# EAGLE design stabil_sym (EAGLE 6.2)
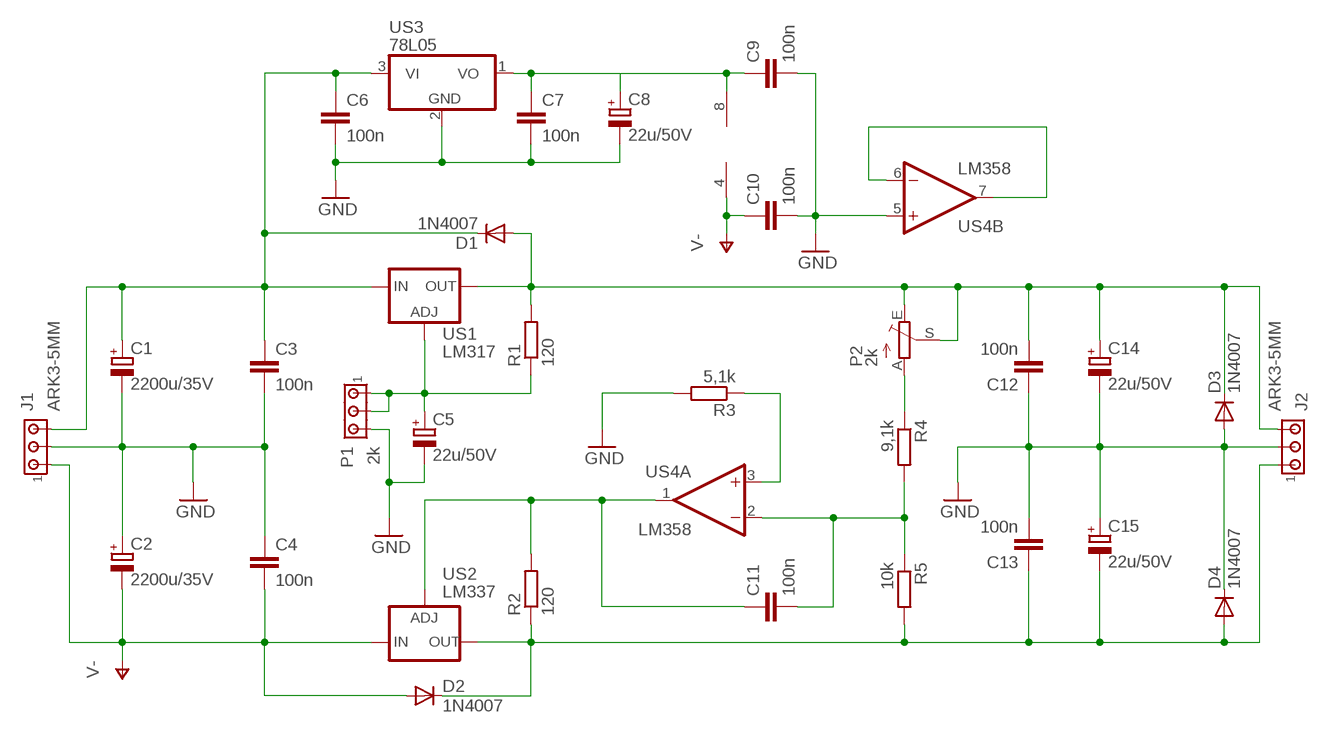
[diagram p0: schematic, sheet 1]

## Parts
C1  2200u/35V  CPOL-EUE7.5-18  [E7,5-18]
C2  2200u/35V  CPOL-EUE7.5-18  [E7,5-18]
C3  100n  C-EU050-025X075  [C050-025X075]
C4  100n  C-EU050-025X075  [C050-025X075]
C5  22u/50V  CPOL-EUE2.5-6  [E2,5-6]
C6  100n  C-EU050-025X075  [C050-025X075]
C7  100n  C-EU050-025X075  [C050-025X075]
C8  22u/50V  CPOL-EUE2.5-6  [E2,5-6]
C9  100n  C-EU050-025X075  [C050-025X075]
C10  100n  C-EU050-025X075  [C050-025X075]
C11  100n  C-EU050-025X075  [C050-025X075]
C12  100n  C-EU050-025X075  [C050-025X075]
C13  100n  C-EU050-025X075  [C050-025X075]
C14  22u/50V  CPOL-EUE2.5-6  [E2,5-6]
C15  22u/50V  CPOL-EUE2.5-6  [E2,5-6]
D1  1N4007  1N4004  [DO41-10]
D2  1N4007  1N4004  [DO41-10]
D3  1N4007  1N4004  [DO41-10]
D4  1N4007  1N4004  [DO41-10]
J1  ARK3-5MM  [3PIN-5MM]
J2  ARK3-5MM  [3PIN-5MM]
P1  2k  ARK3-5MM  [3PIN-5MM]
P2  2k  TRIM_EU-B64Y  [B64Y]
R1  120  R-EU_0207/7  [0207/7]
R2  120  R-EU_0207/7  [0207/7]
R3  5,1k  R-EU_0207/7  [0207/7]
R4  9,1k  R-EU_0207/7  [0207/7]
R5  10k  R-EU_0207/7  [0207/7]
US1  LM317  LM317TS  [317TS]
US2  LM337  LM337TS  [337TS]
US3  78L05  7805L  [TO92]
US4  LM358  LM358N  [DIL08]

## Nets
GND: C1.- C2.+ C3.2 C4.1 C5.- C6.2 C7.2 C8.- C9.2 C10.2 C12.1 C13.2 C14.- C15.+ D3.A D4.C J1.P$2 J2.P$2 P1.P$3 R3.2 US3.2(GND) US4.5(B:+IN)
N$1: C1.+ C3.1 C6.1 D1.C J1.P$3 US1.3(IN) US3.3(VI)
N$2: R3.1 US4.3(A:+IN)
N$3: P2.A R4.1
N$4: C12.2 C14.+ D1.A D3.C J2.P$3 P2.E P2.S R1.2 US1.2(OUT)
N$5: C13.1 C15.- D2.C D4.A J2.P$1 R2.1 R5.2 US2.3(OUT)
N$6: C5.+ P1.P$1 P1.P$2 R1.1 US1.1(ADJ)
N$7: C11.1 R2.2 US2.1(ADJ) US4.1(A:OUT)
N$8: C11.2 R4.2 R5.1 US4.2(A:-IN)
N$9: C7.1 C8.+ C9.1 US3.1(VO) US4.8(P:V+)
N$10: US4.6(B:-IN) US4.7(B:OUT)
V-: C2.- C4.2 C10.1 D2.A J1.P$1 US2.2(IN) US4.4(P:V-)

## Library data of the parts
C1 C2 C5 C8 C14 C15 = rcl:CPOL-EU: POLARIZED CAPACITOR, European symbol
C3 C4 C6 C7 C9-C13 = rcl:C-EU: CAPACITOR, European symbol
D1-D4 = diode:1N4004: DIODE
J1 J2 P1 = zlacza_futrzak:ARK3: ARK 3 Raster 5mm i 3,5mm
P2 = pot:TRIM_EU-: POTENTIOMETER
R1-R5 = rcl:R-EU_: RESISTOR, European symbol
US1 = v-reg:LM317TS: VOLTAGE REGULATOR
US2 = v-reg:LM337TS: VOLTAGE REGULATOR
US3 = linear:78*: Positive VOLTAGE REGULATOR Source: http://cache.national.com/ds/LM/LM78L05.pdf http://www.fairchildsemi.com/ds/LM/LM7805.pdf
US4 = linear:LM358: OP AMP also LM158; LM258; LM2904 Source: http://cache.national.com/ds/LM/LM158.pdf

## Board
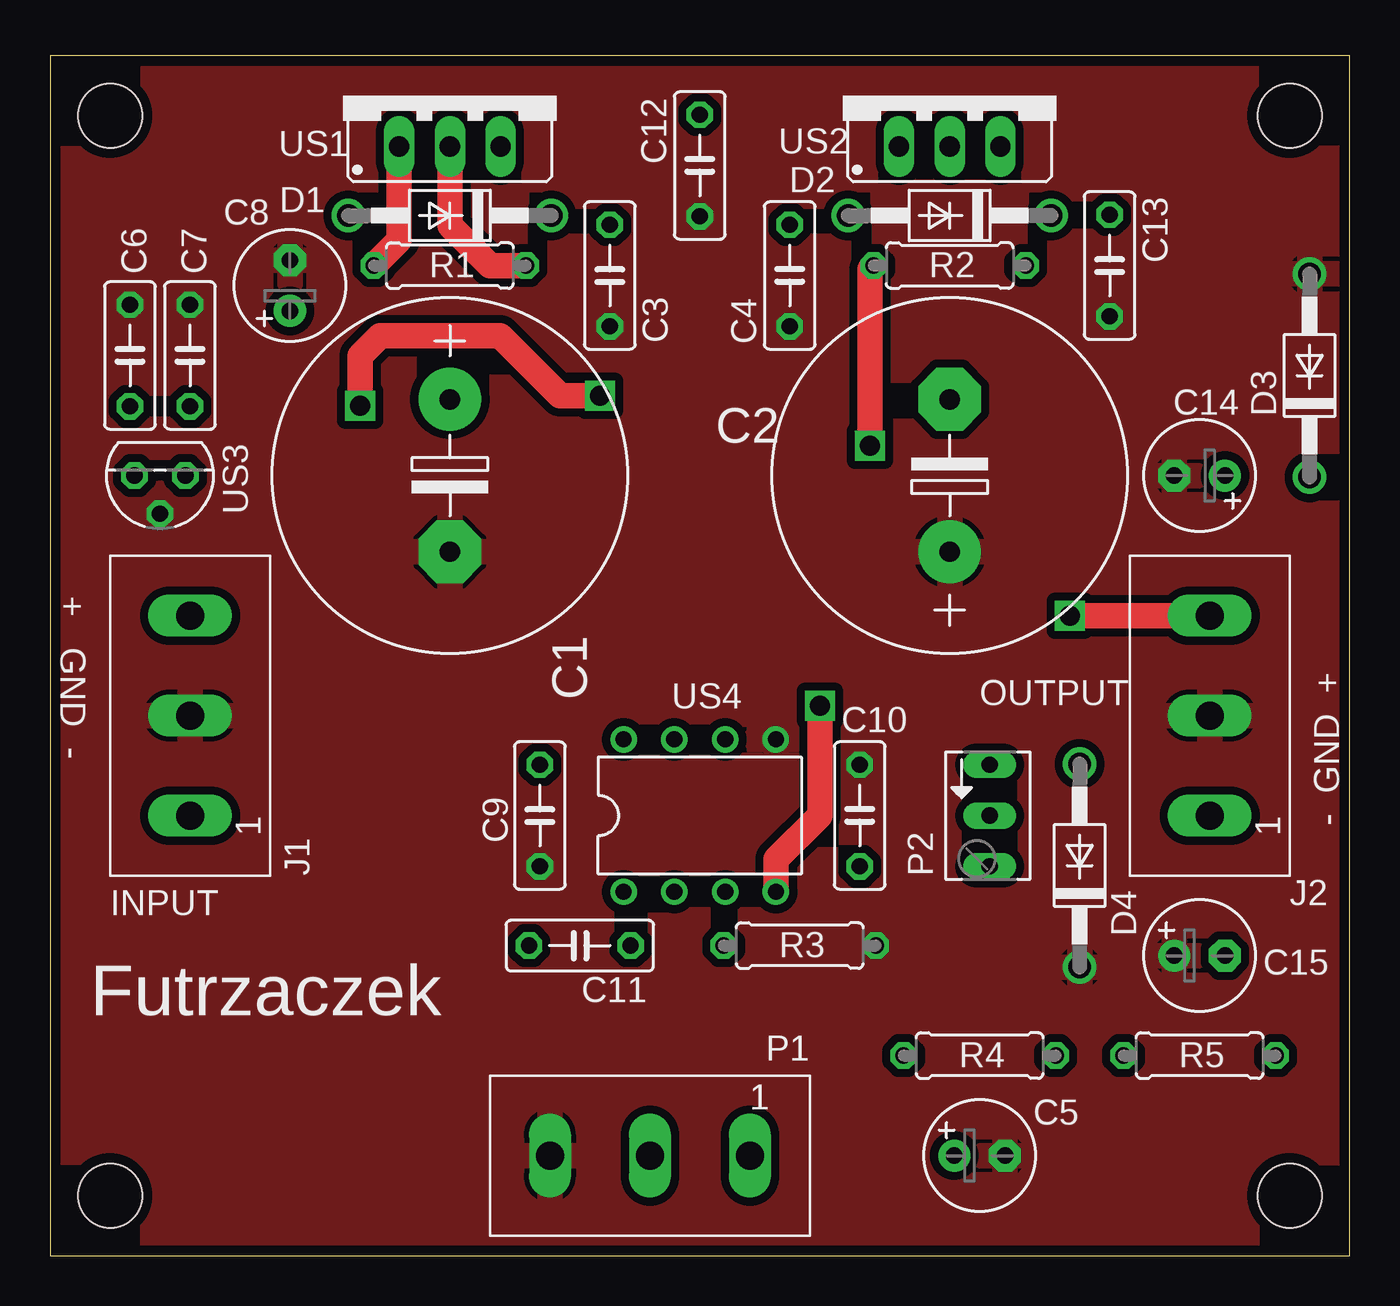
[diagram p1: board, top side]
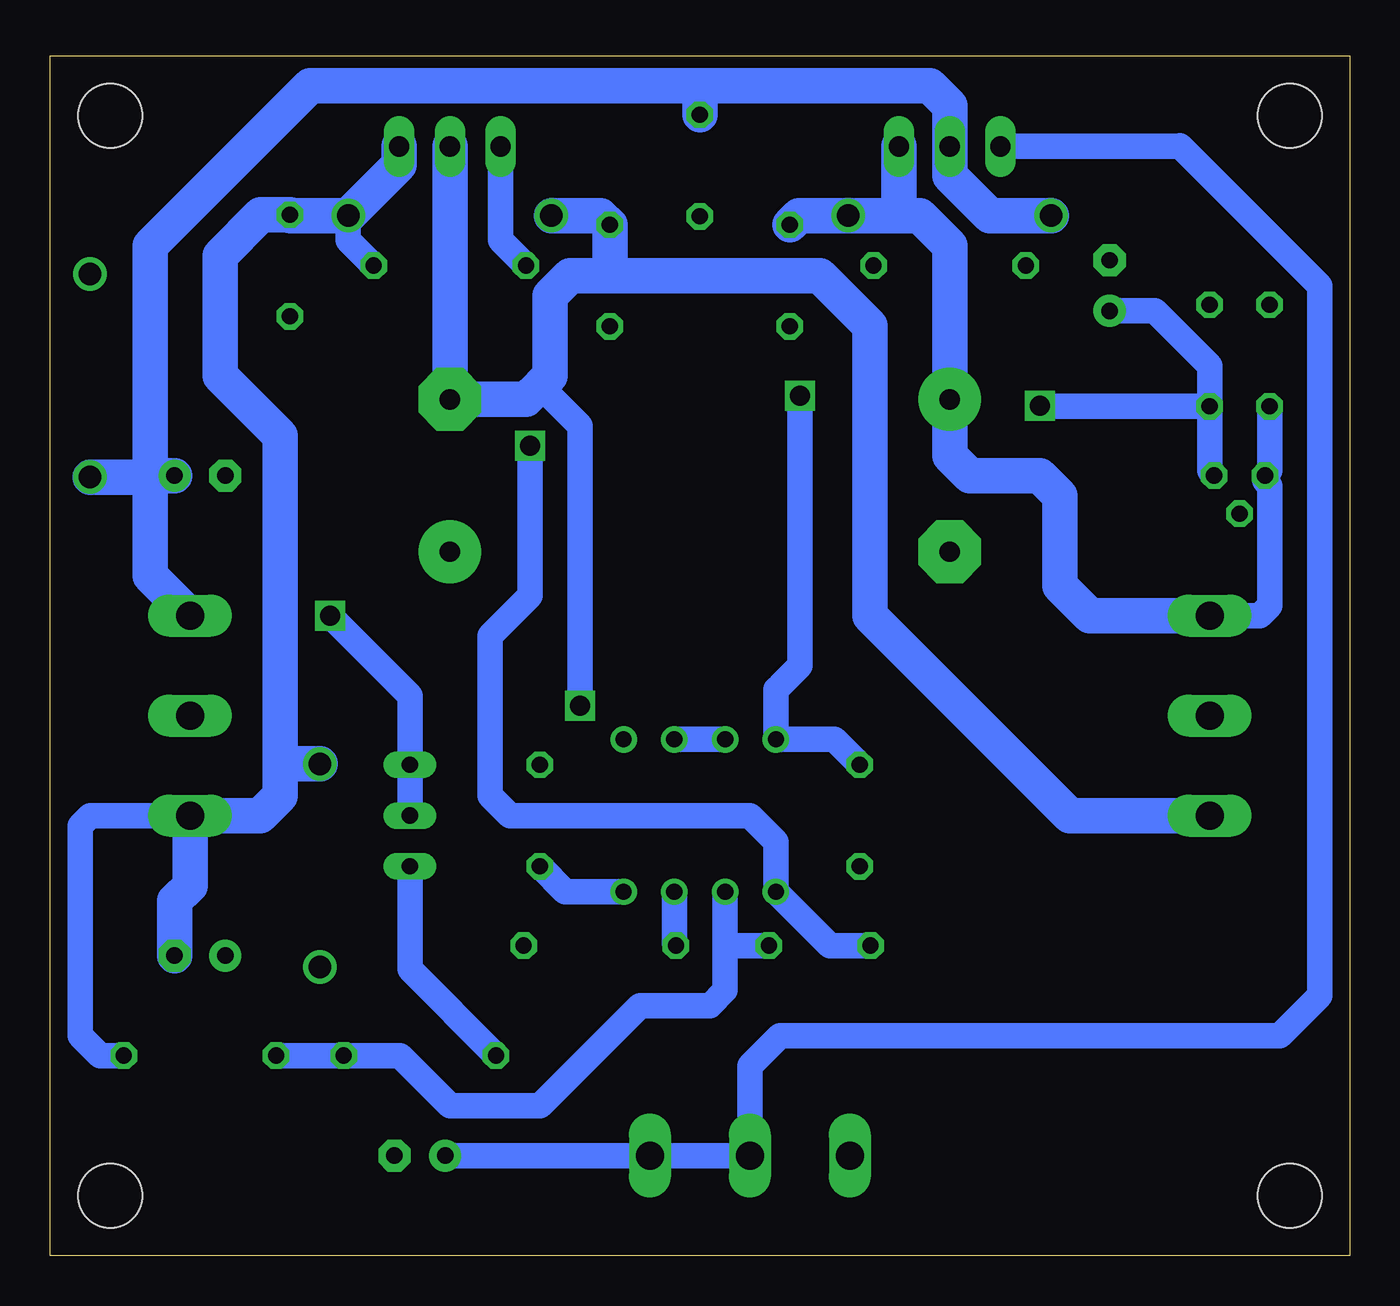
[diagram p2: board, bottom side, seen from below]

Size 65 x 60 mm. Coordinates in mm from the lower left corner, seen from the top.
Outline: 0,0 65,0 65,60 0,60 0,0
Copper layers (1*16): Top 0.035mm / dielectric 1.5mm / Bottom 0.035mm
Design rules: minimum track width 10mil, minimum drill 23mil, track to track 8mil, track to pad 8mil, pad to pad 8mil, via to via 8mil, smd to smd 8mil, copper to edge 20mil, drill to drill 8mil, minimum pad ring 10mil, minimum via ring 8mil, stop-mask expansion 4mil, vias tented up to drill 0mil, thermal gap 10mil
Holes 3.2 mm at 3,3 3,57 62,3 62,57

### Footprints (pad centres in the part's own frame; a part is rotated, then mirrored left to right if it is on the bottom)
E7,5-18 = drill 1.016 pad 3.15: + -3.81,0 | drill 1.016 pad 3.15 octagon: - 3.81,0
C050-025X075 = drill 0.813 octagon: 1 -2.54,0; 2 2.54,0
E2,5-6 = drill 0.813 pad 1.6: + -1.27,0 | drill 0.813 pad 1.6 octagon: - 1.27,0
DO41-10 = drill 1.118: A 5.08,0; C -5.08,0
3PIN-5MM = drill 1.4 long: P$1 -5,0; P$2 0,0; P$3 5,0
B64Y = drill 0.813 long: A 2.54,0; E -2.54,0; S 0,0
0207/7 = drill 0.813 octagon: 1 -3.81,0; 2 3.81,0
317TS = drill 1.016 long: 1 -2.54,-2.54; 2 0,-2.54; 3 2.54,-2.54
337TS = drill 1.016 long: 1 -2.54,-2.54; 2 0,-2.54; 3 2.54,-2.54
TO92 = drill 0.813 octagon: 1 -1.27,0; 2 0,1.905; 3 1.27,0
DIL08 = drill 0.813 pad 1.27: 1 -3.81,-3.81; 2 -1.27,-3.81; 3 1.27,-3.81; 4 3.81,-3.81; 5 3.81,3.81; 6 1.27,3.81; 7 -1.27,3.81; 8 -3.81,3.81

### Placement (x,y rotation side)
C1  20,39 270 top
C2  45,39 90 top
C3  28,49 270 top
C4  37,49 90 top
C5  46.5,5 0 top
C6  4,45 90 top
C7  7,45 90 top
C8  12,48.5 90 top
C9  24.5,22 270 top
C10  40.5,22 90 top
C11  26.5,15.5 0 top
C12  32.5,54.5 90 top
C13  53,49.5 270 top
C14  57.5,39 180 top
C15  57.5,15 0 top
D1  20,52 180 top
D2  45,52 180 top
D3  63,44 90 top
D4  51.5,19.5 90 top
J1  7,27 90 top
J2  58,27 90 top
P1  30,5 180 top
P2  47,22 270 top
R1  20,49.5 0 top
R2  45,49.5 180 top
R3  37.5,15.5 0 top
R4  46.5,10 0 top
R5  57.5,10 0 top
US1  20,58 0 top
US2  45,58 0 top
US3  5.5,39 180 top
US4  32.5,22 0 top

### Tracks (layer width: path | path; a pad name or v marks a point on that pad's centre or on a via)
GND
  pour Top (isolate 0.406): 0,0 65,0 65,60 0,60
N$1
  Bottom 1.27: C6.1 4,39.23 US3.3 4.23,38.73 4,38.5 4,32.5 4.5,32 J1.P$3
  Bottom 1.778: 8,32 J1.P$3 13,32 14.5,33.5 14.5,38 15.5,39 19,39 20,40 C1.+ 20,50.5 21.5,52 22.5,52 | 22.5,52 D1.C 27.54,52 C3.1 | US1.3 22.54,52.04 22.5,52
N$2
  Bottom 1.27: US4.3 33.77,15.58 R3.1
N$3
  Bottom 1.27: P2.A 47,14.31 R4.1
N$4  (via drill 1)
  Top 1.27: US1.2 20,51.5 21.5,50 22,49.5 R1.2 | v51,32 J2.P$3
  Bottom 1.27: P2.S P2.E 47,27 47,28 v51,32
  Bottom 1.778: 32.5,58.5 29.5,58.5 25,58.5 21,58.5 20,57.5 US1.2 20,54.5 20,54 18,52 15.5,52 D1.A | 32.5,58.5 52,58.5 60,50.5 60,39 | C12.2 32.5,58.5 | C14.+ 60,39 | D3.C 60.08,38.92 60,39 | 60,39 60,34 J2.P$3
N$5
  Bottom 1.27: D2.C 50.08,50.77 R2.1 | R5.2 62.5,10 63.5,11 63.5,21.5 63,22 J2.P$1
  Bottom 1.778: US2.3 47.54,54.54 D2.C 52.96,52 C13.1 54.46,52.04 56.5,50 56.5,44 53.5,41 53.5,25.5 53.5,24.5 | 53.5,24.5 53.5,23 54.5,22 J2.P$1 58,18.5 58.77,17.73 C15.- | D4.A 53.42,24.58 53.5,24.5
N$6
  Top 1.27: US1.1 17.46,51.27 17.46,50.77 R1.1
  Bottom 1.27: C5.+ P1.P$1 P1.P$2 30,9.5 28.5,11 3.5,11 1.5,13 1.5,32 1.5,48.5 8.5,55.5 8.54,55.46 US1.1
N$7  (via drill 1)
  Top 1.27: v41,40.5 41,49.31 R2.2
  Bottom 1.27: US2.1 42.46,50.77 R2.2 | v41,40.5 41,33 43,31 43,23 42,22 30,22 28.69,20.69 US4.1 26,15.5 C11.1
N$8
  Bottom 1.27: US4.2 31.23,15.5 | 31.23,15.5 31.23,13.27 32,12.5 35.5,12.5 40.5,7.5 45,7.5 47.5,10 R4.2 R5.1 | C11.2 31.23,15.5
N$9  (via drill 1)
  Top 1.27: v27.5,43 25.5,43 22.5,46 16.5,46 15.5,45 v15.5,42.5
  Bottom 1.27: C8.+ 9.73,47.23 9.5,47 7,44.5 C7.1 | C9.1 25.77,25.81 US4.8 28.69,28.31 28.5,28.5 27.5,29.5 v27.5,43 | C7.1 15.46,42.46 v15.5,42.5 | C7.1 7,39.23 US3.1
N$10
  Bottom 1.27: US4.7 US4.6
V-  (via drill 1)
  Top 1.27: US4.4 36.31,19.81 38.5,22 v38.5,27.5
  Bottom 1.27: US4.4 39.23,18.19 C10.1 | v38.5,27.5 38.5,41.5 40.5,43.5
  Bottom 1.778: US2.2 C2.- 41.19,42.81 40.5,43.5 40,44 40,48 39,49 37,49 | 37,49 26.5,49 24,46.5 24,41 24,34 24,32 17.25,25.25 14,22 12,22 J1.P$1 | 37,49 C4.2 37.46,52 D2.A

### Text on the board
tPlace: + GND - | OUTPUT | - GND + | INPUT | Futrzaczek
